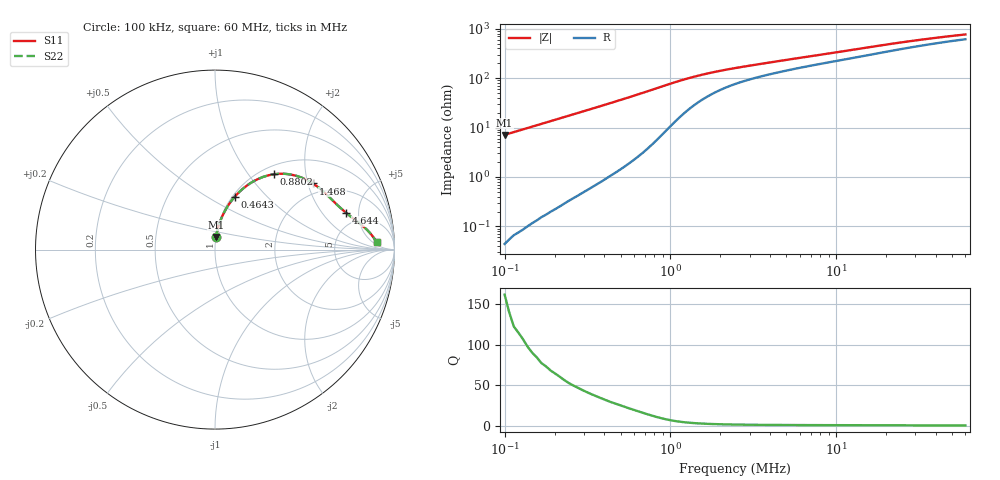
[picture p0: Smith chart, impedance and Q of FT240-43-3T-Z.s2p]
! ListType=Log
!!FT240-43 3T Z
# MHZ S RI R 50
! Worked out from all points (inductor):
!   101 points, 100 kHz to 60 MHz, reference 50 ohm
!   read as one part in series: L = 11.3 uH near 100 kHz
!   highest Q = 161 at 100 kHz (marker M1), where L = 11.3 uH
!   S11 on the Smith chart (normalised r, x): 100 kHz: 1.00, +0.14; 464.3 kHz: 1.03, +0.67; 880.2 kHz: 1.14, +1.34; 1.468 MHz: 1.65, +2.15; 4.644 MHz: 3.73, +3.60; 60 MHz: 16, +7
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0.1  0.00598 0.0708  0.995 -0.0709  0.995 -0.0708  0.00598 0.0707
0.1376916  0.0111 0.0969  0.99 -0.097  0.99 -0.097  0.011 0.0968
0.1778417  0.018 0.1241  0.9831 -0.1244  0.9831 -0.1244  0.0179 0.124
0.2296993  0.0293 0.1584  0.9717 -0.1588  0.9717 -0.1587  0.0293 0.1584
0.2966783  0.0478 0.2008  0.9532 -0.2013  0.9533 -0.2012  0.0476 0.2007
0.3831879  0.0772 0.2517  0.9236 -0.2523  0.9238 -0.2522  0.0771 0.2515
0.4642547  0.1101 0.2946  0.8907 -0.2954  0.8908 -0.2952  0.11 0.2944
0.5624719  0.1558 0.3396  0.845 -0.3405  0.8452 -0.3404  0.1555 0.3394
0.6392399  0.1951 0.3688  0.8056 -0.3698  0.8058 -0.3697  0.1948 0.3687
0.7744768  0.2692 0.4054  0.7314 -0.4066  0.7317 -0.4066  0.2689 0.4053
0.8801799  0.3279 0.4198  0.6726 -0.4211  0.673 -0.4211  0.3275 0.4198
1.06639  0.4202 0.4186  0.5802 -0.42  0.5805 -0.4202  0.4199 0.4188
1.291994  0.5014 0.3928  0.4988 -0.3943  0.4989 -0.3945  0.5012 0.393
1.46833  0.5448 0.3687  0.4552 -0.3702  0.4554 -0.3704  0.5447 0.3689
1.896486  0.6093 0.3187  0.3907 -0.3203  0.3908 -0.3205  0.6092 0.3189
2.611302  0.6626 0.2667  0.3372 -0.2685  0.3372 -0.2686  0.6626 0.2667
4.643984  0.7325 0.2037  0.2671 -0.2063  0.2671 -0.2063  0.7324 0.2037
7.267103  0.7771 0.1676  0.2224 -0.1712  0.2224 -0.1713  0.777 0.1676
12.92394  0.826 0.129  0.1731 -0.135  0.1731 -0.135  0.826 0.1291
21.55992  0.86 0.0964  0.1388 -0.1058  0.1388 -0.1059  0.86 0.0964
38.34252  0.8862 0.0637  0.1123 -0.0801  0.1123 -0.0801  0.8862 0.0638
60  0.9006 0.0409  0.0974 -0.0662  0.0974 -0.0662  0.9008 0.0412
